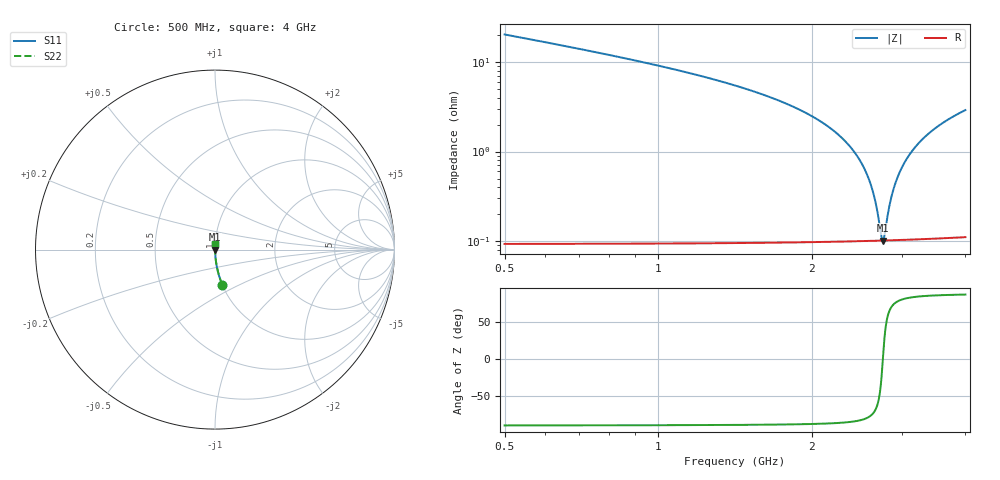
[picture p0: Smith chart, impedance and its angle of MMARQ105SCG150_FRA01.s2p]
! MMARQ105SCG150_FRA01  S-PARAMETER MODEL  ( General Type )
! Model Generated by TAIYO YUDEN Corporation (http://www.ty-top.com)
! Version 1.0
! TAIYO YUDEN Control No. 200326
! Copyright(c) 2020 TAIYO YUDEN CO.,LTD. All Rights Reserved.
! Product Description (link to TY-COMPAS)
! https://ds.yuden.co.jp/TYCOMPAS/or/detail?pn=MMARQ105SCG150JFRA01&u=M
! Products Name : Multilayer Ceramic Capacitors
! Characteristics :
!  Capacitance : 15 pF , Rated Voltage : 250V , TCC : CG / C0G
!  Case Size : 1.0 x 0.5 / 0.039 x 0.02 [mm/inch] , Thickness : 0.5 / 0.02 [mm/inch]
!  (Conditions: Temperature = 25 degC , DC Bias Current/Voltage = 0A / 0V)
! External Node Assignments :
!  1  o---| |---o  2
! GND o---------o GND
! Frequency Range : 500MHz  -  4GHz  [ 401 STEP ]
# MHz S RI R 50
! Freq[MHz].  S11 Real  S11 Imag  S21 Real  S21 Imag  S12 Real  S12 Imag  S22 Real  S22 Imag
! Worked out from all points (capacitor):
!   401 points, 500 MHz to 4 GHz, reference 50 ohm
!   read as one part in series: C = 15.1 pF near 517.5 MHz
!   lowest |Z| = 102 mohm at 2.757 GHz (marker M1)
!   series resonance near 2.756 GHz, so ESL is about 220 pH
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500  0.0405 -0.195  0.9595 0.195  0.9595 0.195  0.0405 -0.195
762.5  0.0168 -0.1251  0.9832 0.1251  0.9832 0.1251  0.0168 -0.1251
1086.25  0.00756 -0.0811  0.9924 0.0811  0.9924 0.0811  0.00756 -0.0811
1672.5  0.00253 -0.0396  0.9975 0.0396  0.9975 0.0396  0.00253 -0.0396
2005  0.00158 -0.0246  0.9984 0.0246  0.9984 0.0246  0.00158 -0.0246
2250  0.00123 -0.0156  0.9988 0.0156  0.9988 0.0156  0.00123 -0.0156
2433.75  0.00108 -0.00949  0.9989 0.00949  0.9989 0.00949  0.00108 -0.00949
2565  0.00103 -0.00547  0.999 0.00547  0.999 0.00547  0.00103 -0.00547
2643.75  0.00102 -0.00317  0.999 0.00317  0.999 0.00317  0.00102 -0.00317
2678.75  0.00101 -0.00217  0.999 0.00217  0.999 0.00217  0.00101 -0.00217
2731.25  0.00101 -0.000689  0.999 0.000689  0.999 0.000689  0.00101 -0.000689
2748.75  0.00101 -0.000202  0.999 0.000202  0.999 0.000202  0.00101 -0.000202
2757.5  0.00101 3.96e-05  0.999 -3.96e-05  0.999 -3.96e-05  0.00101 3.96e-05
2775  0.00101 0.000521  0.999 -0.000521  0.999 -0.000521  0.00101 0.000521
2836.25  0.00102 0.00218  0.999 -0.00218  0.999 -0.00218  0.00102 0.00218
2880  0.00103 0.00335  0.999 -0.00335  0.999 -0.00335  0.00103 0.00335
2923.75  0.00104 0.0045  0.999 -0.0045  0.999 -0.0045  0.00104 0.0045
3037.5  0.00109 0.00741  0.9989 -0.00741  0.9989 -0.00741  0.00109 0.00741
3203.75  0.00118 0.0115  0.9988 -0.0115  0.9988 -0.0115  0.00118 0.0115
3422.5  0.00134 0.0166  0.9987 -0.0166  0.9987 -0.0166  0.00134 0.0166
3685  0.00158 0.0224  0.9984 -0.0224  0.9984 -0.0224  0.00158 0.0224
4000  0.00195 0.029  0.9981 -0.029  0.9981 -0.029  0.00195 0.029
